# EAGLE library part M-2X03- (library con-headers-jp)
MALE HEADER
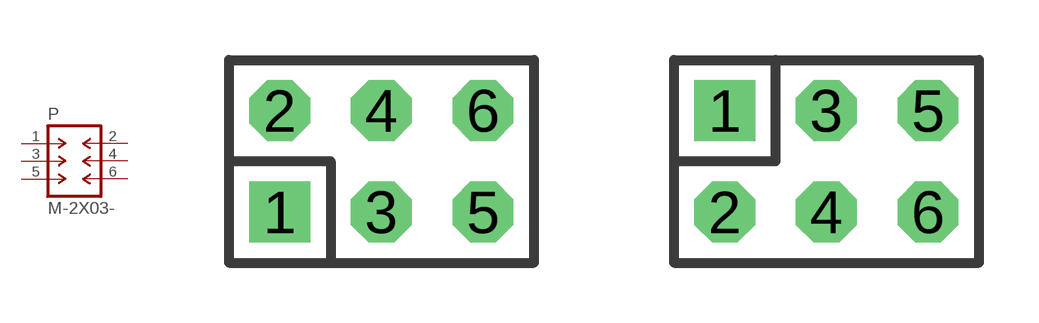
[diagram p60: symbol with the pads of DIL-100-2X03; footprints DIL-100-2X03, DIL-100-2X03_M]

Designator prefix P

## M-2X03-DIL-100  [DIL-100-2X03]
1  1  pas
2  2  pas
3  3  pas
4  4  pas
5  5  pas
6  6  pas

## M-2X03-DIL-100_M  [DIL-100-2X03_M]
Pads as for DIL-100-2X03

## M-2X03-DIL-2MM  [DIL-2MM-2X03]
Pads as for DIL-100-2X03

## M-2X03-DIL-2MM_M  [DIL-2MM-2X03_M]
Pads as for DIL-100-2X03

## Footprint DIL-100-2X03 (pad centres in mm)
PIN HEADER - 0.1"
drill 1.016 square: 1 -2.54,-1.27
drill 1.016 octagon: 2 -2.54,1.27; 3 0,-1.27; 4 0,1.27; 5 2.54,-1.27; 6 2.54,1.27

## Footprint DIL-100-2X03_M (pad centres in mm)
PIN HEADER - MIRRORED 0.1"
drill 1.016 square: 1 -2.54,1.27
drill 1.016 octagon: 2 -2.54,-1.27; 3 0,1.27; 4 0,-1.27; 5 2.54,1.27; 6 2.54,-1.27

## Footprint DIL-2MM-2X03 (pad centres in mm)
PIN HEADER - 2MM"
drill 0.711 square: 1 -2,-1
drill 0.711: 2 -2,1; 3 0,-1; 4 0,1; 5 2,-1; 6 2,1

## Footprint DIL-2MM-2X03_M (pad centres in mm)
PIN HEADER - MIRRORED 2MM
drill 0.711 square: 1 -2,1
drill 0.711: 2 -2,-1; 3 0,1; 4 0,-1; 5 2,1; 6 2,-1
